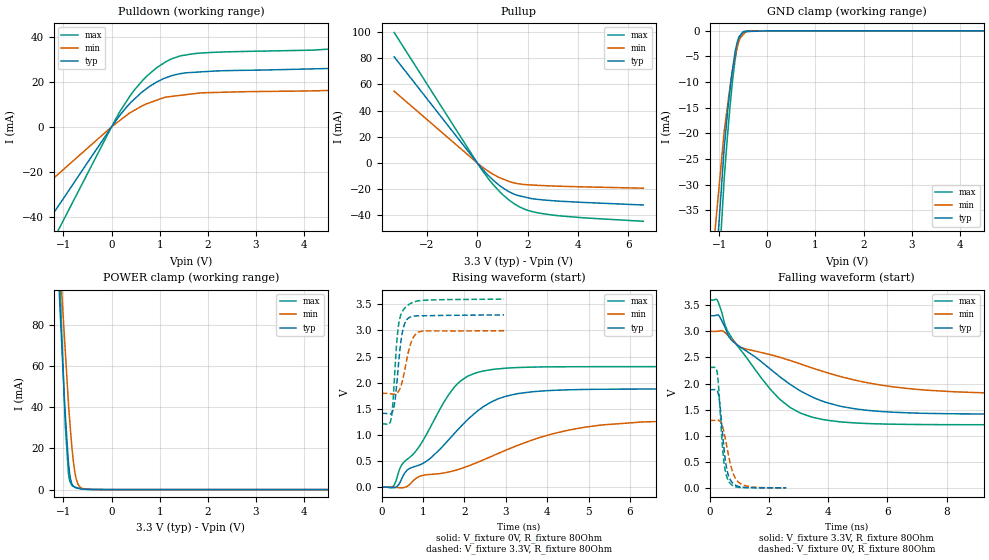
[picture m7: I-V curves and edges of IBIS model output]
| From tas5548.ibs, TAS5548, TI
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|   output Model
[Model]   output
Model_type   3-state
Polarity   Non-Inverting
Vmeas = 1.65
Vref = 1.65
Cref = 2pF
Rref = 80
|   typ   min   max
|   (nom PVT)   (fast PVT)   (slow PVT)
|C_comp from frequency sweep method (F=50MHz)
|C_comp   3.021e-12   2.837e-12   3.231e-12
|ON state : BUFFER OUTPUT TURNED HIGH
|C_comp   3.021e-12   2.837e-12   3.231e-12
|OFF state: BUFFER IN HIGH IMPEDANCE
|C_comp   1.399e-12   1.380e-12   1.405e-12
|C_comp from LC tank measurement(L=1nH)
|Resonant Frequency(Hz)   4.410e+09   4.450e+09   4.380e+09
C_comp   1.304e-12   1.280e-12   1.322e-12
|ON state : BUFFER OUTPUT TURNED HIGH
|Resonant Frequency(Hz)   4.410e+09   4.450e+09   4.380e+09
|C_comp   1.304e-12   1.280e-12   1.322e-12
|OFF state: BUFFER IN HIGH IMPEDANCE
|Resonant Frequency(Hz)   4.580e+09   4.640e+09   4.530e+09
|C_comp   1.209e-12   1.178e-12   1.236e-12
| Where nom  PVT is Nominal Process, 3.3V, 27C
|   Fast PVT is Strong Process,  3.6V, 0C
|   Slow PVT is Weak Process,   3V, 125C
[Voltage Range]   3.3   3   3.6
|Ambient Temperature   27   125   0
|Junction Temperature
[Temperature Range]   27   125   0
[Pullup Reference]   3.3   3   3.6
[Pulldown Reference]   0   0   0
[Power Clamp Reference]   3.3   3   3.6
[GND Clamp Reference]   0   0   0
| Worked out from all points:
|   slope of the pulldown table from 0 to 0.495 V, typ, clamps not added: 38.8 ohm
|   slope of the pullup table from 0 to 0.495 V, typ, clamps not added: 46.9 ohm
|   GND clamp passes 1 mA (typ) near -0.57 V on its own axis
|   POWER clamp passes 1 mA (typ) near -0.76 V on its own axis
|   falling waveform, V_fixture 3.3V, R_fixture 80Ohm: 20-80 % time 2.67ns typ, 4.23ns min, 1.87ns max; typ from 3.3 V to 1.41 V
|   rising waveform, V_fixture 0V, R_fixture 80Ohm: 20-80 % time 1.67ns typ, 2.82ns min, 1.17ns max; typ from 0 V to 1.88 V
|   rising waveform, V_fixture 3.3V, R_fixture 80Ohm: 20-80 % time 149ps typ, 203ps min, 133ps max; typ from 1.41 V to 3.3 V
|   falling waveform, V_fixture 0V, R_fixture 80Ohm: 20-80 % time 211ps typ, 310ps min, 176ps max; typ from 1.88 V to 0.002 V
[Pulldown]
|   Voltage   I(typ)   I(min)   I(max)
-3.3V     -104.8mA   -62.36mA   -136.8mA
-132mV    -4.193mA   -2.494mA   -5.472mA
172.8mV   5.184mA    2.866mA    6.814mA
478.8mV   12.43mA    7.439mA    16.49mA
939.6mV   19.95mA    11.89mA    26.32mA
1.246V    22.75mA    13.56mA    30.23mA
1.829V    24.43mA    15.06mA    32.79mA
4.162V    25.79mA    16.03mA    34.12mA
5.174V    27.87mA    17.42mA    36.98mA
5.726V    31.62mA    19.38mA    41.9mA
6V        34.91mA    21.05mA    46.09mA
6.6V      44.69mA    24.71mA    58.92mA
[GND Clamp]
|   Voltage   I(typ)   I(min)   I(max)
-3.3V     -1.709A    -1.468A    -1.81A
-1.544V   -110mA     -85.26mA   -132.1mA
-897.6mV  -22.79mA   -19.55mA   -28.81mA
-818.4mV  -14.95mA   -13.88mA   -19.29mA
-781.2mV  -11.83mA   -11.22mA   -15.2mA
-745.8mV  -8.871mA   -8.967mA   -11.79mA
-680.4mV  -4.695mA   -5.443mA   -6.285mA
-633.6mV  -2.465mA   -3.447mA   -3.438mA
-594mV    -1.265mA   -2.104mA   -1.792mA
-501.6mV  -162.9uA   -723.1uA   -245.3uA
-285mV    -92.11uA   -4.021uA   -18.91uA
6.6V      0A         0A         0A
[Pullup]
|   Voltage   I(typ)   I(min)   I(max)
-3.3V     80.99mA    54.74mA    99.56mA
172.8mV   -4.03mA    -2.652mA   -5.005mA
633.6mV   -13.2mA    -8.722mA   -16.61mA
939.6mV   -18.01mA   -11.65mA   -22.92mA
1.278V    -22.12mA   -14.3mA    -28.6mA
1.554V    -24.58mA   -15.65mA   -32.17mA
1.912V    -26.18mA   -16.57mA   -35.59mA
2.473V    -28mA      -17.19mA   -38.35mA
4.162V    -30.11mA   -18.27mA   -41.84mA
6.6V      -32.14mA   -19.3mA    -44.59mA
[POWER Clamp]
|   Voltage   I(typ)   I(min)   I(max)
-3.3V     1.403A     1.109A     1.949A
-1.082V   93.36mA    113.8mA    109.3mA
-1.051V   78.18mA    101.8mA    86.25mA
-1.048V   76.44mA    100.4mA    83.77mA
-961.2mV  36.26mA    67.07mA    30.92mA
-896.4mV  13.19mA    42.14mA    7.987mA
-838.2mV  3.718mA    24.52mA    2.709mA
-795mV    1.688mA    14mA       1.612mA
-745.8mV  880uA      6.417mA    1.162mA
-660mV    419.1uA    1.28mA     613.4uA
-333mV    113uA      4.542uA    10.36uA
6.6V      0A         0A         0A
[Ramp]
R_load = 80
|   typ   min   max
dV/dt_r   1.12794/1.66725e-09   0.775713/2.81255e-09   1.38391/1.17091e-09
dV/dt_f   1.13316/2.65958e-09   0.722426/4.23112e-09   1.43407/1.87081e-09
[Falling Waveform]
V_fixture = 3.3V
V_fixture_min = 3V
V_fixture_max = 3.6V
R_fixture = 80Ohm
|   Time   V(typ)   V(min)   V(max)
0s        3.3V       3V         3.6V
252ps     3.313V     3.001V     3.604V
648ps     2.9V       2.903V     2.963V
1.052ns   2.691V     2.695V     2.638V
2.06ns    2.271V     2.551V     1.882V
2.696ns   1.992V     2.445V     1.55V
3.416ns   1.753V     2.307V     1.363V
4.892ns   1.517V     2.067V     1.246V
7.1ns     1.431V     1.883V     1.215V
15ns      1.411V     1.796V     1.21V
[Rising Waveform]
V_fixture = 0V
V_fixture_min = 0V
V_fixture_max = 0V
R_fixture = 80Ohm
|   Time   V(typ)   V(min)   V(max)
0s        1.666nV    35.53nV    1.383nV
288ps     -12.04mV   232.3uV    28.16mV
484ps     167mV      -11.8mV    428.1mV
640ps     343mV      30.35mV    549.6mV
900ps     421.6mV    203.4mV    772mV
1.756ns   1.029V     318.4mV    1.916V
2.436ns   1.53V      516.2mV    2.221V
3.304ns   1.793V     806.5mV    2.29V
5.332ns   1.875V     1.192V     2.306V
15ns      1.88V      1.293V     2.307V
[Rising Waveform]
V_fixture = 3.3V
V_fixture_min = 3V
V_fixture_max = 3.6V
R_fixture = 80Ohm
|   Time   V(typ)   V(min)   V(max)
0s        1.411V     1.795V     1.21V
224ps     1.406V     1.785V     1.3V
268ps     1.462V     1.779V     1.597V
316ps     1.638V     1.78V      2.198V
396ps     2.273V     1.825V     3.044V
480ps     2.878V     1.976V     3.335V
580ps     3.173V     2.337V     3.447V
724ps     3.265V     2.803V     3.527V
900ps     3.279V     2.972V     3.568V
2.956ns   3.297V     2.994V     3.598V
[Falling Waveform]
V_fixture = 0V
V_fixture_min = 0V
V_fixture_max = 0V
R_fixture = 80Ohm
|   Time   V(typ)   V(min)   V(max)
0s        1.88V      1.293V     2.307V
256ps     1.859V     1.3V       2.199V
336ps     1.643V     1.283V     1.643V
412ps     1.194V     1.214V     942.4mV
472ps     817.9mV    1.096V     542.7mV
572ps     379.8mV    810.9mV    224.3mV
660ps     198.6mV    559.2mV    111.7mV
836ps     65.59mV    219.9mV    28.23mV
1.072ns   13.36mV    73.01mV    8.899mV
2.58ns    1.988mV    2.715mV    1.393mV
